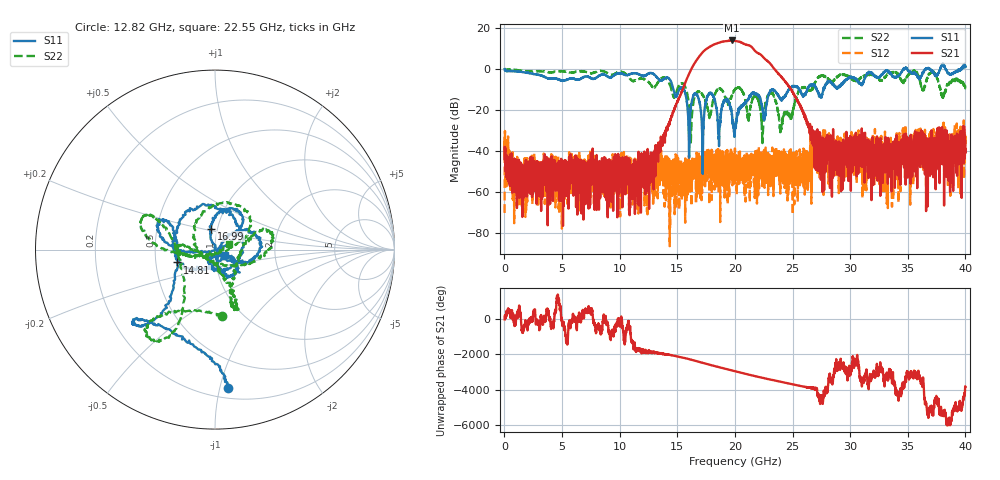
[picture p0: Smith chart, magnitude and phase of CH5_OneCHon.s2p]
!Keysight Technologies,N5245B,MY57181321,A.14.80.03
!Date: Thursday, March 28, 2024 19:42:14
!Correction: S11(C  2-Port  )
!S21(C  2-Port  )
!S12(C  2-Port  )
!S22(C  2-Port  )
!S2P File: Measurements: S11, S21, S12, S22:
# Hz S  RI  R 50
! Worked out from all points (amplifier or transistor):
!   4000 points, 10 MHz to 40 GHz, reference 50 ohm
!   highest |S21| = 13.8 dB at 19.73 GHz (marker M1)
!   |S21| within 3 dB of that: 17.85 GHz to 21.42 GHz (3.573 GHz wide, 18.2 % of centre)
!   unconditionally stable (mu >= 1): start of sweep to 34.63 GHz; 34.96 GHz to 36.56 GHz; 38.26 GHz to 39.61 GHz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
!   at 6.67 GHz: K = 16755.15, MAG = -43.6 dB, |S12| = -55.4 dB
!   at 20.01 GHz: K = 44.88, MAG = 14.1 dB, |S12| = -53.6 dB
!   at 40 GHz: K = -536.67, MSG = -2.5 dB, |S12| = -34.0 dB
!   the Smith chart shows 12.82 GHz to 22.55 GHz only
!   S11 on the Smith chart (normalised r, x): 12.82 GHz: 0.27, -1.06; 14.81 GHz: 0.65, -0.10; 16.99 GHz: 0.93, +0.22; 22.55 GHz: 1.12, -0.07
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1e7  0.9885 -0.0648  0.0118 -0.0043  5.51e-06 -0.000311  -0.9472 0.0853
6.68e9  0.2935 0.5058  0.000184 0.00024  0.000731 0.00117  0.8118 0.3362
1.282e10  0.0713 -0.7733  0.000216 -0.00582  0.00238 -0.00128  0.0371 -0.3692
1.334e10  -0.0691 -0.5696  -0.0102 -0.00624  -0.00595 -0.00246  -0.3034 -0.3734
1.481e10  -0.2091 -0.0714  0.0292 0.1097  -0.00395 0.00409  -0.2227 0.014
1.616e10  0.0913 0.0443  -0.5565 -0.7342  0.000779 -0.00125  -0.0083 -0.0182
1.699e10  -0.0209 0.1172  0.2126 2.162  -0.00378 0.00261  0.0826 0.2586
1.752e10  0.1493 -0.0775  3.017 -0.5151  -0.00268 0.00411  -0.1158 0.0692
1.799e10  0.2299 0.0768  -0.0886 -3.674  -0.000164 0.000624  0.077 -0.0886
1.858e10  0.0346 0.00883  -4.245 0.7737  -0.00054 -0.000892  0.3139 0.0562
1.913e10  0.0962 -0.1406  0.794 4.621  0.003 -0.00484  0.1973 0.062
1.946e10  0.1247 -0.0918  4.4 2.043  0.00251 0.00478  0.1215 -0.0683
1.973e10  0.0698 -0.0306  4.64 -1.644  0.00103 0.00392  0.0926 -0.2041
2.001e10  0.000363 -0.0344  2.012 -4.336  -0.00184 0.000998  0.0946 -0.3036
2.063e10  0.0569 -0.1122  -4.14 -1.227  -0.00398 0.000465  0.1038 -0.2639
2.122e10  0.1143 0.1615  -0.574 3.683  0.00284 -0.000659  -0.0614 -0.0354
2.178e10  -0.2081 0.1256  2.614 0.6276  0.00132 -0.00327  -0.2189 0.00304
2.255e10  0.056 -0.0323  -0.2721 -1.789  0.0105 -0.00224  0.0795 0.0323
2.357e10  -0.1579 0.2162  -0.3845 0.8086  0.0061 0.0114  -0.0146 0.1489
2.667e10  0.1415 0.3812  0.000384 0.0389  0.000972 -0.000304  0.0129 0.3257
3.334e10  0.4486 0.7139  -0.00201 0.0116  0.00833 -0.00411  0.7439 -0.2005
4e10  0.9197 0.6515  -0.00895 0.00666  0.0117 0.0162  0.00558 -0.3391
